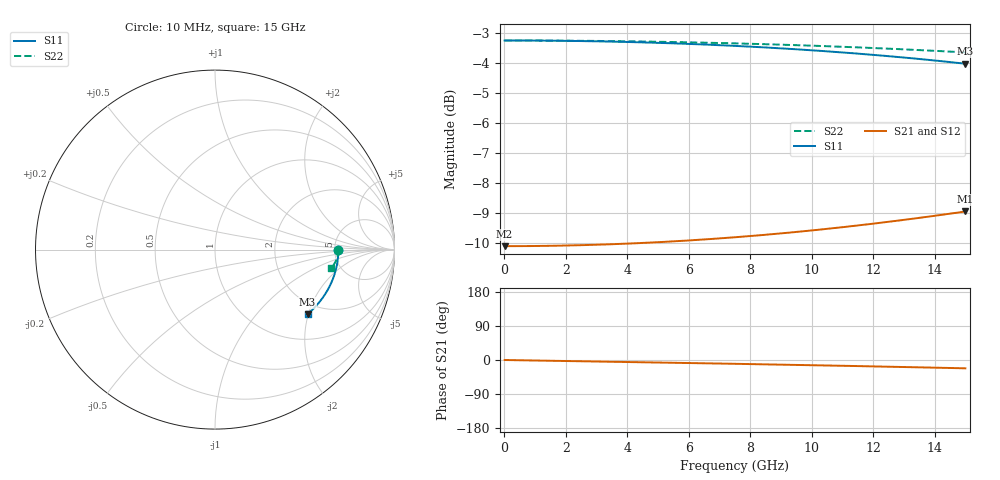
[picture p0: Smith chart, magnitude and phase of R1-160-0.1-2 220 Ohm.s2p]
!version-1
!date-03.2021
# MHz S RI R 50
!Freq ReS11 ImS11 ReS21 ImS21 ReS12 ImS12 ReS22 ImS22
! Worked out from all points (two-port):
!   751 points, 10 MHz to 15 GHz, reference 50 ohm
!   highest |S21| = -8.95 dB at 15 GHz (marker M1); lowest = -10.1 dB at 10 MHz (marker M2)
!   |S21| within 3 dB of the highest: start of sweep to end of sweep
!   lowest |S11| = -4.0 dB at 15 GHz (marker M3), VSWR 4.39, Z = 83 - j98.9 ohm
!   |S11| at or under -10 dB: nowhere
!   |S22| runs from -3.7 to -3.3 dB; largest |S21 - S12| = 0
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10  0.6875 -0.000251  0.3125 -7.07e-05  0.3125 -7.07e-05  0.6875 -6.96e-05
70  0.6875 -0.00176  0.3125 -0.000495  0.3125 -0.000495  0.6875 -0.000487
1270  0.6864 -0.0319  0.3127 -0.009  0.3127 -0.009  0.6872 -0.00883
2510  0.683 -0.063  0.3132 -0.0179  0.3132 -0.0179  0.6864 -0.0174
3770  0.6774 -0.0946  0.3141 -0.0271  0.3141 -0.0271  0.6851 -0.0262
5010  0.6696 -0.1255  0.3152 -0.0364  0.3152 -0.0364  0.6832 -0.0348
5650  0.6647 -0.1414  0.3159 -0.0414  0.3159 -0.0414  0.6821 -0.0392
6270  0.6593 -0.1567  0.3167 -0.0463  0.3167 -0.0463  0.6808 -0.0435
6890  0.6533 -0.172  0.3175 -0.0513  0.3175 -0.0513  0.6794 -0.0478
7510  0.6468 -0.1872  0.3184 -0.0564  0.3184 -0.0564  0.6779 -0.052
8150  0.6394 -0.2028  0.3194 -0.0619  0.3194 -0.0619  0.6762 -0.0564
8770  0.6316 -0.2178  0.3204 -0.0673  0.3204 -0.0673  0.6744 -0.0607
9390  0.6231 -0.2328  0.3214 -0.0729  0.3214 -0.0729  0.6724 -0.0649
10010  0.614 -0.2476  0.3225 -0.0787  0.3225 -0.0787  0.6704 -0.0691
10650  0.604 -0.2627  0.3236 -0.0849  0.3236 -0.0849  0.6681 -0.0735
11270  0.5935 -0.2772  0.3247 -0.0911  0.3247 -0.0911  0.6657 -0.0777
11890  0.5824 -0.2915  0.3258 -0.0975  0.3258 -0.0975  0.6632 -0.0819
12510  0.5706 -0.3057  0.327 -0.1041  0.327 -0.1041  0.6606 -0.0861
13110  0.5584 -0.3191  0.328 -0.1108  0.328 -0.1108  0.6579 -0.0902
13690  0.5461 -0.3319  0.329 -0.1175  0.329 -0.1175  0.6552 -0.0941
14610  0.5251 -0.3517  0.3305 -0.1286  0.3305 -0.1286  0.6506 -0.1003
15000  0.5157 -0.3599  0.331 -0.1335  0.331 -0.1335  0.6486 -0.1029
